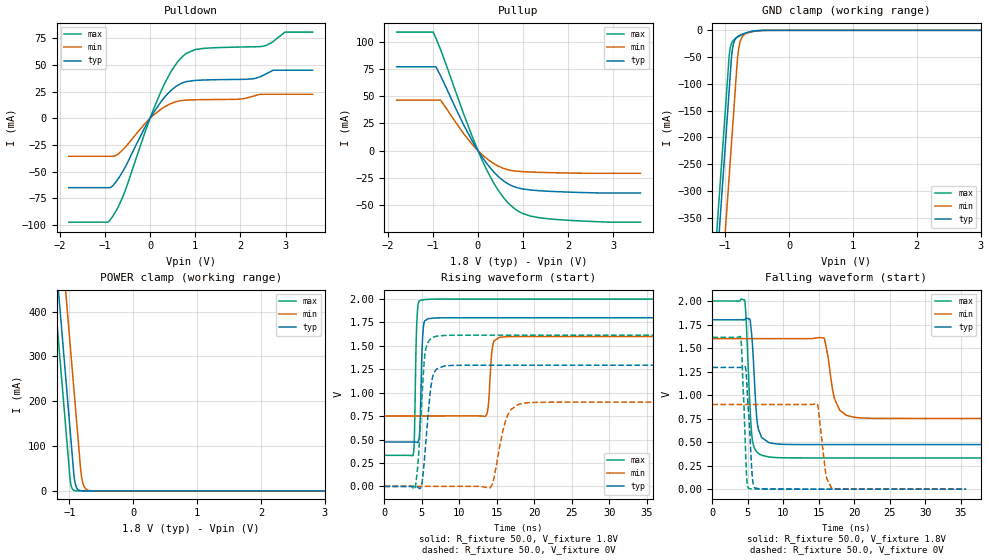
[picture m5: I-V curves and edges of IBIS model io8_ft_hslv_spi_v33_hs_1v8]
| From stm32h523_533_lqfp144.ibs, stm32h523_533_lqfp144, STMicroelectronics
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[Model]   io8_ft_hslv_spi_v33_hs_1v8
Model_type I/O
Polarity   Non-Inverting
Enable   Active-Low
| CAP_THRESHOLD on pad IOFT is "UDTCAPC" :
| Rising=20.0% of vddiom   Falling=80.0% of vddiom
| C_comp min and max val. don't necessarily correlate with the min and max pvt
| but are the smallest and greatest pad capacitance found.
| var   typ   min   max
C_comp   3.69208pF  3.66980pF  3.86736pF
|C_comp_pullup   2.29895pF  2.22605pF  2.22535pF
|C_comp_pulldown   1.39313pF  1.44375pF  1.64201pF
Vinl = 480.0mV
Vinh = 1.4V
Vmeas = 900.0mV   | Reference voltage for timing measurements
Cref  = 50.0pF   | Timing specification test load capacitance value
Rref  = 100.0MOhm   | Timing specification test load resistance value
Vref  = 900.0mV   | Timing specification test load voltage
[Model Spec]
| TIME_THRESHOLD on pin ZIV33M is "CMOS" :
| Rising=40.0% of vddiom   Falling=60.0% of vddiom
Vinl 693.80000mV 621.80000mV 774.80000mV
Vinh 1.05820V 933.20000mV 1.16320V
| variable   typ   min   max
[Temperature Range] 25.0 125.0 -40.0
| variable   typ   min   max
[Voltage Range] 1.8V 1.6V 2.0V
| variable   typ   min   max
[POWER Clamp Reference] 1.8V 1.6V 2.0V
| variable   typ   min   max
[GND Clamp Reference] 0V 0V 0V
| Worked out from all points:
|   slope of the pulldown table from 0 to 0.27 V, typ, clamps not added: 15.8 ohm
|   slope of the pullup table from 0 to 0.27 V, typ, clamps not added: 17.1 ohm
|   GND clamp passes 1 mA (typ) near -0.52 V on its own axis
|   POWER clamp passes 1 mA (typ) near -0.84 V on its own axis
|   rising waveform, R_fixture 50.0, V_fixture 1.8V: 20-80 % time 275ps typ, 413ps min, 247ps max; typ from 0.474 V to 1.8 V
|   falling waveform, R_fixture 50.0, V_fixture 1.8V: 20-80 % time 635ps typ, 1.21ns min, 618ps max; typ from 1.8 V to 0.474 V
|   rising waveform, R_fixture 50.0, V_fixture 0V: 20-80 % time 850ps typ, 1.42ns min, 722ps max; typ from 0 V to 1.29 V
|   falling waveform, R_fixture 50.0, V_fixture 0V: 20-80 % time 590ps typ, 817ps min, 491ps max; typ from 1.29 V to 0 V
[POWER Clamp]
-1.8V     1.518A     1.709A     1.407A
-1.23V    548.8mA    740.2mA    437.5mA
-1.16V    429.8mA    621.2mA    318.5mA
-1.05V    242.8mA    434.2mA    131.5mA
-980mV    123.8mA    315.2mA    17.95mA
-930mV    38.81mA    230.2mA    1.49mA
-910mV    17.82mA    196.2mA    550.8uA
-890mV    8.18mA     162.2mA    203.5uA
-810mV    363.5uA    33.6mA     3.797uA
-770mV    76.62uA    10.47mA    518.8nA
-710mV    7.416uA    1.822mA    26.33nA
3.6V      0A         0A         0A
[GND Clamp]
-1.8V     -1.579A    -1.74A     -1.515A
-1.24V    -627.3mA   -788.3mA   -562.7mA
-1.05V    -304.3mA   -465.3mA   -239.7mA
-940mV    -117.3mA   -278.3mA   -52.69mA
-930mV    -100.3mA   -261.3mA   -40.52mA
-900mV    -50.11mA   -210.3mA   -24.23mA
-880mV    -30.95mA   -176.3mA   -20.02mA
-810mV    -12.18mA   -57.97mA   -13.23mA
-780mV    -9.807mA   -29.1mA    -11.19mA
-690mV    -5.41mA    -7.142mA   -6.184mA
-420mV    -170.4uA   -446.1uA   -81.94uA
3.6V      5.755nA    953.2nA    228.2pA
| variable   typ   min   max
[Pullup Reference] 1.8V 1.6V 2.0V
| variable   typ   min   max
[Pulldown Reference] 0V 0V 0V
[Pullup]
-1.8V     77.07mA    46.37mA    109mA
-990mV    77.07mA    46.37mA    109mA
-930mV    77.07mA    46.37mA    103.2mA
-830mV    68.91mA    46.37mA    93.11mA
-310mV    23.14mA    15.23mA    32.99mA
120mV     -7.558mA   -4.734mA   -11.27mA
460mV     -24.18mA   -14.48mA   -37.09mA
630mV     -29.66mA   -17.24mA   -46.33mA
800mV     -33.21mA   -18.68mA   -53.07mA
1.18V     -36.34mA   -19.79mA   -60.45mA
1.56V     -37.44mA   -20.28mA   -62.79mA
3.6V      -39.03mA   -20.93mA   -65.9mA
[Pulldown]
-1.8V     -65.02mA   -35.56mA   -97.42mA
-940mV    -65.02mA   -35.56mA   -97.42mA
-850mV    -64.17mA   -35.56mA   -93.49mA
-570mV    -47.32mA   -28.01mA   -70.04mA
-120mV    -9.088mA   -5.279mA   -14.07mA
250mV     16.04mA    8.832mA    26.05mA
550mV     29.17mA    15.25mA    49.41mA
780mV     34.17mA    17.07mA    60.14mA
1.18V     35.97mA    17.56mA    65.65mA
2.49V     40mA       22.62mA    67.56mA
2.99V     45.21mA    22.62mA    80.94mA
3.6V      45.21mA    22.62mA    80.94mA
[Ramp]
dV/dt_r 776.15658mV/848.19317ps 539.56193mV/1.41422ns 968.54178mV/716.98775ps
dV/dt_f 795.78703mV/633.75213ps 508.98054mV/1.11945ns 1.00099V/616.93673ps
R_load = 50.0
| Removed startup time: 0s 0s 0s  .
| Removed end time: 35.75ns.
[Rising Waveform]
R_fixture   = 50.0
V_fixture   = 1.8V
V_fixture_min = 1.6V
V_fixture_max = 2.0V
0s        473.7mV    751.7mV    331.7mV
3.85ns    473.7mV    751.7mV    341.9mV
4.3ns     471.2mV    751.7mV    1.714V
4.75ns    656mV      751.7mV    1.984V
5.15ns    1.654V     751.7mV    1.992V
5.85ns    1.791V     751.7mV    1.997V
13.45ns   1.8V       746.4mV    2V
14.45ns   1.8V       1.5V       2V
15.35ns   1.8V       1.592V     2V
35.75ns   1.8V       1.6V       2V
| Removed startup time: 0s 0s 0s  .
| Removed end time: 48.75ns.
[Falling Waveform]
R_fixture   = 50.0
V_fixture   = 1.8V
V_fixture_min = 1.6V
V_fixture_max = 2.0V
0s        1.8V       1.6V       2V
4.55ns    1.8V       1.6V       2.011V
5.3ns     1.806V     1.6V       877.2mV
5.6ns     1.588V     1.6V       545.4mV
6.25ns    764.6mV    1.6V       397.6mV
6.95ns    548.6mV    1.6V       360.1mV
15.75ns   473.7mV    1.604V     331.7mV
17.2ns    473.7mV    963.6mV    331.7mV
18.9ns    473.7mV    784.3mV    331.7mV
48.75ns   473.7mV    751.7mV    331.7mV
| Removed startup time: 0s 0s 0s  .
| Removed end time: 48.7ns.
[Rising Waveform]
R_fixture   = 50.0
V_fixture   = 0V
V_fixture_min = 0V
V_fixture_max = 0V
0s        180.7nV    438nV      126.8nV
4.1ns     384.6uV    438.3nV    -22.17mV
4.9ns     -2.559mV   424.5nV    797.1mV
5.4ns     346mV      410nV      1.41V
6.1ns     996.6mV    381.9nV    1.569V
6.6ns     1.208V     355.3nV    1.595V
14.1ns    1.293V     -14.9mV    1.614V
16.2ns    1.294V     707.8mV    1.614V
17.9ns    1.294V     876.8mV    1.614V
48.7ns    1.294V     899.3mV    1.614V
| Removed startup time: 0s 0s 0s  .
| Removed end time: 35.75ns.
[Falling Waveform]
R_fixture   = 50.0
V_fixture   = 0V
V_fixture_min = 0V
V_fixture_max = 0V
0s        1.294V     899.3mV    1.614V
4ns       1.294V     899.3mV    1.608V
4.8ns     1.201V     899.3mV    174.7mV
5.15ns    771.2mV    899.3mV    8.324mV
5.6ns     156.9mV    899.3mV    3.01mV
5.95ns    14.34mV    899.3mV    2.183mV
14.75ns   28.21uV    907.7mV    11.08uV
16ns      19.86uV    156.7mV    6.919uV
16.8ns    15.99uV    10.53mV    5.179uV
35.75ns   152nV      11.08uV    31.97nV
